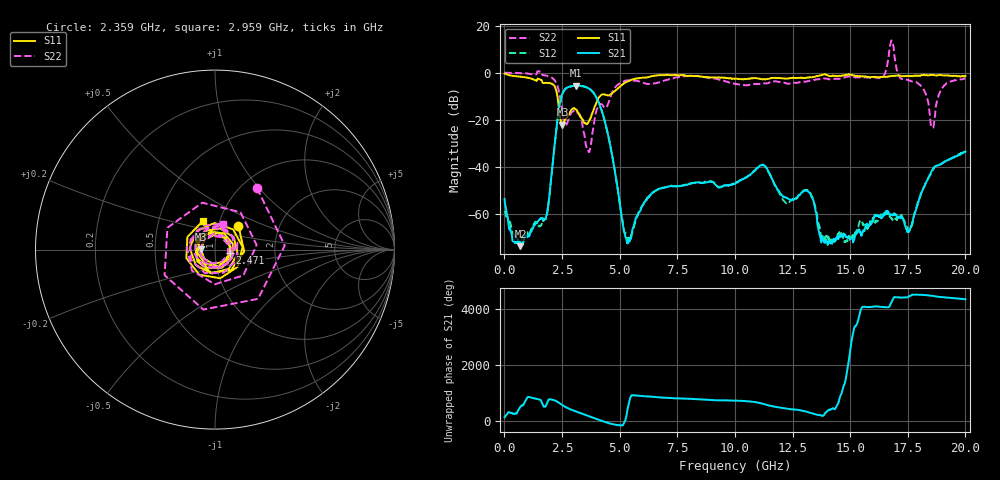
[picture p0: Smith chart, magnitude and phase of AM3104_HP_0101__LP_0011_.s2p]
!Created with skrf (http://scikit-rf.org).
# Hz S RI R 50.0
!freq ReS11 ImS11 ReS21 ImS21 ReS12 ImS12 ReS22 ImS22
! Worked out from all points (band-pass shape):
!   1601 points, 10 MHz to 20 GHz, reference 50 ohm
!   highest |S21| = -5.49 dB at 3.121 GHz (marker M1); lowest = -73.7 dB at 697.2 MHz (marker M2)
!   |S21| within 3 dB of the highest: 2.537 GHz to 3.863 GHz (1.326 GHz wide, 41.4 % of centre)
!   lowest |S11| = -22.1 dB at 2.521 GHz (marker M3), VSWR 1.17, Z = 42.8 + j0.234 ohm
!   |S11| at or under -10 dB: 2.3 GHz to 4.146 GHz (1.846 GHz wide, 57.3 % of centre)
!   |S22| runs from -33.8 to 13.7 dB; largest |S21 - S12| = 0.029
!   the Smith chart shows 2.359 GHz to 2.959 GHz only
!   S11 on the Smith chart (normalised r, x): 2.359 GHz: 1.25, +0.34; 2.471 GHz: 1.18, -0.04; 2.959 GHz: 0.83, +0.27
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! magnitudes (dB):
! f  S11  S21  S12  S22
! 10 MHz  -0.4  -53.7  -58.7  0.0
! 697.2 MHz  -1.7  -73.7  -71.8  -0.2
! 1.809 GHz  -4.3  -61.4  -61.6  -1.3
! 2.359 GHz  -14.7  -15.9  -15.9  -7.6
! 2.471 GHz  -21.3  -10.3  -10.3  -13.4
! 2.521 GHz  -22.1  -8.8  -8.9  -16.8
! 2.959 GHz  -15.3  -5.6  -5.7  -16.4
! 3.121 GHz  -15.7  -5.5  -5.5  -16.9
! 3.346 GHz  -19.4  -5.6  -5.7  -20.1
! 3.658 GHz  -20.8  -6.7  -6.8  -33.6
! 4.27 GHz  -9.2  -17.6  -17.6  -13.9
! 5.332 GHz  -3.8  -72.5  -70.6  -3.2
! 6.682 GHz  -1.1  -49.5  -49.5  -4.2
! 10.01 GHz  -2.7  -47.3  -46.9  -4.8
! 11.2 GHz  -2.8  -39.1  -39.2  -4.6
! 13.34 GHz  -2.0  -52.9  -52.4  -3.3
! 14.12 GHz  -1.4  -72.2  -70.9  -2.8
! 16.68 GHz  -1.5  -60.2  -60.6  7.2
! 17.56 GHz  -1.4  -67.3  -67.0  -3.4
! 18.56 GHz  -0.9  -41.3  -41.6  -23.4
! 19.01 GHz  -1.1  -38.5  -38.3  -6.3
! 20 GHz  -1.4  -33.6  -33.3  -2.5
